|   stm32f401_d_e_ufbga100 IBIS Model
[IBIS ver]   4.2
[File name]  stm32f401_d_e_ufbga100.ibs
[File Rev]   1.0
[Date]   09-06-2015
[Source] Data Created at STMicroelectronics
[Notes]   File originated from ELDO simulations.
[Disclaimer]  This information is for modeling purpose only and is
   not guaranted. The information is subject to change without
   notice.
[Copyright] Copyright 2015 STMicroelectronics Inc.
[Component] stm32f401_d_e_ufbga100
[Manufacturer] STMicroelectronics
[Package]
| variable   typ   min   max
R_pkg   0.0   NA   NA
L_pkg   0.0H   NA   NA
C_pkg   0.0F   NA   NA
[Pin]   signal_name   model_name   R_pin   L_pin   C_pin
B2 PE2 io8p_arsudq_ft
A1 PE3 io8p_arsudq_ft
B1 PE4 io8p_arsudq_ft
C2 PE5 io8p_arsudq_ft
D2 PE6 io8p_arsudq_ft
D3 VSS GND
C4 VDD POWER
E2 VBAT POWER
C1 PC13-ANTI_TAMP io8p_arwsudq_ft_v33
D1 PC14-OSC32_IN io8p_arwsudq_ft
E1 PC15-OSC32_OUT io8p_arsudq_ft
F2 VSS GND
G2 VDD POWER
F1 PH0-OSC_IN io8p_arsudq_ft
G1 PH1-OSC_OUT io8p_arsudq_ft
H2 NRST ioreset_ft_v33
H1 PC0 io8p_arwsudq_ft
J2 PC1 io8p_arwsudq_ft
J3 PC2 io8p_arwsudq_ft
K2 PC3 io8p_arwsudq_ft
J1 VSSA GND
K1 VREF- GND
L1 VREF+ POWER
M1 VDDA POWER
L2 PA0-WKUP io8p_arwsudq_ft_v33
M2 PA1 io8p_arwsudq_ft
K3 PA2 io8p_arwsudq_ft
L3 PA3 io8p_arwsudq_ft
E3 BYPASS_REG NC
M3 PA4 io8p_ar3wsudq_ft
K4 PA5 io8p_ar3wsudq_ft
L4 PA6 io8p_ar3wsudq_ft
M4 PA7 io8p_arwsudq_ft
K5 PC4 io8p_arwsudq_ft
L5 PC5 io8p_arwsudq_ft
M5 PB0 io8p_ar3wsudq_ft
M6 PB1 io8p_ar3wsudq_ft
L6 PB2 io8p_arwsudq_ft
M7 PE7 io8p_arwsudq_ft
L7 PE8 io8p_arwsudq_ft
M8 PE9 io8p_arwsudq_ft
L8 PE10 io8p_arwsudq_ft
M9 PE11 io8p_arwsudq_ft
L9 PE12 io8p_arsudq_ft
M10 PE13 io8p_arsudq_ft
M11 PE14 io8p_arsudq_ft
M12 PE15 io8p_ar3wsudq_ft
L10 PB10 io8p_arsudq_i2cin_ft
K9 PB11 io8p_arsudq_ft
L11 VCAP1 POWER
F12 VSS GND
G12 VDD POWER
L12 PB12 io8p_arsudq_ft
K12 PB13 io8p_arsudq_ft
K11 PB14 io8p_arsudq_ft
K10 PB15 io8p_arsudq_ft
K8 PD9 io8p_arsudq_ft
J12 PD10 io8p_arsudq_ft
J11 PD11 io8p_arsudq_ft
J10 PD12 io8p_arsudq_ft
H12 PD13 io8p_arsudq_ft
H11 PD14 io8p_arsudq_ft
H10 PD15 io8p_arsudq_ft
E12 PC6 io8p_arsudq_ft
E11 PC7 io8p_arsudq_ft
E10 PC8 io8p_arsudq_ft
D12 PC9 io8p_arsudq_i2cin_ft
D11 PA8 io8p_arsudq_i2cin_ft
D10 PA9 io8usb_vbus_otg_ft
C12 PA10 io8usb_id_otg_ft
B12 PA11 io8usb_lsfs_otg_ft
A12 PA12 io8usb_lsfs_otg_ft
A11 PA13 io8p_arsudq_ft
C11 VCAP2 POWER
F11 VSS GND
G11 VDD POWER
A10 PA14 io8p_arsudq_ft
A9 PA15 io8p_arsudq_ft
B11 PC10 io8p_arsudq_ft
C10 PC11 io8p_arsudq_ft
B10 PC12 io8p_arsudq_ft
C9 PD0 io8p_arsudq_ft
B9 PD1 io8p_arsudq_ft
C8 PD2 io8p_arsudq_ft
B8 PD3 io8p_arsudq_ft
B7 PD4 io8p_arsudq_ft
A6 PD5 io8p_arsudq_ft
B6 PD6 io8p_arsudq_ft
A5 PD7 io8p_arsudq_ft
A8 PB3 io8p_arsudq_i2cin_ft
A7 PB4 io8p_arsudq_i2cin_ft
C5 PB5 io8p_ar3wsudq_ft
B5 PB6 io8p_arsudq_i2cin_ft
B4 PB7 io8p_arsudq_i2cin_ft
A4 BOOT0 vpp_test_hv
A3 PB8 io8p_arsudq_i2cin_ft
B3 PB9 io8p_arsudq_i2cin_ft
C3 PE0 io8p_arsudq_ft
A2 PE1 io8p_arsudq_ft
H3 PDR_ON NC
[Diff Pin]   inv_pin   vdiff   tdelay_typ  tdelay_min  tdelay_max
B12 A12 200mV   NA   NA   NA
[Model Selector] io8p_ar3wsudq_ft
io8p00_ar3wsudq_ft_pd_lv  "SPEED00 1P8V, PD=40kOhm"
io8p00_ar3wsudq_ft_pu_lv  "SPEED00 1P8V, PU=40kOhm"
io8p00_ar3wsudq_ft_lv  "SPEED00 1P8V"
io8p01_ar3wsudq_ft_pd_lv  "SPEED01 1P8V, PD=40kOhm"
io8p01_ar3wsudq_ft_pu_lv  "SPEED01 1P8V, PU=40kOhm"
io8p01_ar3wsudq_ft_lv  "SPEED01 1P8V"
io8p10_ar3wsudq_ft_pd_lv  "SPEED10 1P8V, PD=40kOhm"
io8p10_ar3wsudq_ft_pu_lv  "SPEED10 1P8V, PU=40kOhm"
io8p10_ar3wsudq_ft_lv  "SPEED10 1P8V"
io8p11_ar3wsudq_ft_pd_lv  "SPEED11 1P8V, PD=40kOhm"
io8p11_ar3wsudq_ft_pu_lv  "SPEED11 1P8V, PU=40kOhm"
io8p11_ar3wsudq_ft_lv  "SPEED11 1P8V"
io8p00_ar3wsudq_ft_pd  "SPEED00, PD=40kOhm"
io8p00_ar3wsudq_ft_pu  "SPEED00, PU=40kOhm"
io8p00_ar3wsudq_ft  "SPEED00"
io8p01_ar3wsudq_ft_pd  "SPEED01, PD=40kOhm"
io8p01_ar3wsudq_ft_pu  "SPEED01, PU=40kOhm"
io8p01_ar3wsudq_ft  "SPEED01"
io8p10_ar3wsudq_ft_pd  "SPEED10, PD=40kOhm"
io8p10_ar3wsudq_ft_pu  "SPEED10, PU=40kOhm"
io8p10_ar3wsudq_ft  "SPEED10"
io8p11_ar3wsudq_ft_pd  "SPEED11, PD=40kOhm"
io8p11_ar3wsudq_ft_pu  "SPEED11, PU=40kOhm"
io8p11_ar3wsudq_ft  "SPEED11"
[Model Selector] io8p_arsudq_ft
io8p00_arsudq_ft_pd_lv  "SPEED00 1P8V, PD=40kOhm"
io8p00_arsudq_ft_pu_lv  "SPEED00 1P8V, PU=40kOhm"
io8p00_arsudq_ft_lv  "SPEED00 1P8V"
io8p01_arsudq_ft_pd_lv  "SPEED01 1P8V, PD=40kOhm"
io8p01_arsudq_ft_pu_lv  "SPEED01 1P8V, PU=40kOhm"
io8p01_arsudq_ft_lv  "SPEED01 1P8V"
io8p10_arsudq_ft_pd_lv  "SPEED10 1P8V, PD=40kOhm"
io8p10_arsudq_ft_pu_lv  "SPEED10 1P8V, PU=40kOhm"
io8p10_arsudq_ft_lv  "SPEED10 1P8V"
io8p11_arsudq_ft_pd_lv  "SPEED11 1P8V, PD=40kOhm"
io8p11_arsudq_ft_pu_lv  "SPEED11 1P8V, PU=40kOhm"
io8p11_arsudq_ft_lv  "SPEED11 1P8V"
io8p00_arsudq_ft_pd  "SPEED00, PD=40kOhm"
io8p00_arsudq_ft_pu  "SPEED00, PU=40kOhm"
io8p00_arsudq_ft  "SPEED00"
io8p01_arsudq_ft_pd  "SPEED01, PD=40kOhm"
io8p01_arsudq_ft_pu  "SPEED01, PU=40kOhm"
io8p01_arsudq_ft  "SPEED01"
io8p10_arsudq_ft_pd  "SPEED10, PD=40kOhm"
io8p10_arsudq_ft_pu  "SPEED10, PU=40kOhm"
io8p10_arsudq_ft  "SPEED10"
io8p11_arsudq_ft_pd  "SPEED11, PD=40kOhm"
io8p11_arsudq_ft_pu  "SPEED11, PU=40kOhm"
io8p11_arsudq_ft  "SPEED11"
[Model Selector] io8p_arsudq_i2cin_ft
io8p00_arsudq_i2cin_ft_pd_lv  "SPEED00 1P8V, PD=40kOhm"
io8p00_arsudq_i2cin_ft_pu_lv  "SPEED00 1P8V, PU=40kOhm"
io8p00_arsudq_i2cin_ft_lv  "SPEED00 1P8V"
io8p01_arsudq_i2cin_ft_pd_lv  "SPEED01 1P8V, PD=40kOhm"
io8p01_arsudq_i2cin_ft_pu_lv  "SPEED01 1P8V, PU=40kOhm"
io8p01_arsudq_i2cin_ft_lv  "SPEED01 1P8V"
io8p10_arsudq_i2cin_ft_pd_lv  "SPEED10 1P8V, PD=40kOhm"
io8p10_arsudq_i2cin_ft_pu_lv  "SPEED10 1P8V, PU=40kOhm"
io8p10_arsudq_i2cin_ft_lv  "SPEED10 1P8V"
io8p11_arsudq_i2cin_ft_pd_lv  "SPEED11 1P8V, PD=40kOhm"
io8p11_arsudq_i2cin_ft_pu_lv  "SPEED11 1P8V, PU=40kOhm"
io8p11_arsudq_i2cin_ft_lv  "SPEED11 1P8V"
io8p00_arsudq_i2cin_ft_pd  "SPEED00, PD=40kOhm"
io8p00_arsudq_i2cin_ft_pu  "SPEED00, PU=40kOhm"
io8p00_arsudq_i2cin_ft  "SPEED00"
io8p01_arsudq_i2cin_ft_pd  "SPEED01, PD=40kOhm"
io8p01_arsudq_i2cin_ft_pu  "SPEED01, PU=40kOhm"
io8p01_arsudq_i2cin_ft  "SPEED01"
io8p10_arsudq_i2cin_ft_pd  "SPEED10, PD=40kOhm"
io8p10_arsudq_i2cin_ft_pu  "SPEED10, PU=40kOhm"
io8p10_arsudq_i2cin_ft  "SPEED10"
io8p11_arsudq_i2cin_ft_pd  "SPEED11, PD=40kOhm"
io8p11_arsudq_i2cin_ft_pu  "SPEED11, PU=40kOhm"
io8p11_arsudq_i2cin_ft  "SPEED11"
[Model Selector] io8p_arwsudq_ft
io8p00_arwsudq_ft_pd_lv  "SPEED00 1P8V, PD=40kOhm"
io8p00_arwsudq_ft_pu_lv  "SPEED00 1P8V, PU=40kOhm"
io8p00_arwsudq_ft_lv  "SPEED00 1P8V"
io8p01_arwsudq_ft_pd_lv  "SPEED01 1P8V, PD=40kOhm"
io8p01_arwsudq_ft_pu_lv  "SPEED01 1P8V, PU=40kOhm"
io8p01_arwsudq_ft_lv  "SPEED01 1P8V"
io8p10_arwsudq_ft_pd_lv  "SPEED10 1P8V, PD=40kOhm"
io8p10_arwsudq_ft_pu_lv  "SPEED10 1P8V, PU=40kOhm"
io8p10_arwsudq_ft_lv  "SPEED10 1P8V"
io8p11_arwsudq_ft_pd_lv  "SPEED11 1P8V, PD=40kOhm"
io8p11_arwsudq_ft_pu_lv  "SPEED11 1P8V, PU=40kOhm"
io8p11_arwsudq_ft_lv  "SPEED11 1P8V"
io8p00_arwsudq_ft_pd  "SPEED00, PD=40kOhm"
io8p00_arwsudq_ft_pu  "SPEED00, PU=40kOhm"
io8p00_arwsudq_ft  "SPEED00"
io8p01_arwsudq_ft_pd  "SPEED01, PD=40kOhm"
io8p01_arwsudq_ft_pu  "SPEED01, PU=40kOhm"
io8p01_arwsudq_ft  "SPEED01"
io8p10_arwsudq_ft_pd  "SPEED10, PD=40kOhm"
io8p10_arwsudq_ft_pu  "SPEED10, PU=40kOhm"
io8p10_arwsudq_ft  "SPEED10"
io8p11_arwsudq_ft_pd  "SPEED11, PD=40kOhm"
io8p11_arwsudq_ft_pu  "SPEED11, PU=40kOhm"
io8p11_arwsudq_ft  "SPEED11"
[Model Selector] io8p_arwsudq_ft_v33
io8p00_arwsudq_ft_v33_pd_lv  "SPEED00 1P8V, PD=40kOhm"
io8p00_arwsudq_ft_v33_pu_lv  "SPEED00 1P8V, PU=40kOhm"
io8p00_arwsudq_ft_v33_lv  "SPEED00 1P8V"
io8p01_arwsudq_ft_v33_pd_lv  "SPEED01 1P8V, PD=40kOhm"
io8p01_arwsudq_ft_v33_pu_lv  "SPEED01 1P8V, PU=40kOhm"
io8p01_arwsudq_ft_v33_lv  "SPEED01 1P8V"
io8p10_arwsudq_ft_v33_pd_lv  "SPEED10 1P8V, PD=40kOhm"
io8p10_arwsudq_ft_v33_pu_lv  "SPEED10 1P8V, PU=40kOhm"
io8p10_arwsudq_ft_v33_lv  "SPEED10 1P8V"
io8p11_arwsudq_ft_v33_pd_lv  "SPEED11 1P8V, PD=40kOhm"
io8p11_arwsudq_ft_v33_pu_lv  "SPEED11 1P8V, PU=40kOhm"
io8p11_arwsudq_ft_v33_lv  "SPEED11 1P8V"
io8p00_arwsudq_ft_v33_pd  "SPEED00, PD=40kOhm"
io8p00_arwsudq_ft_v33_pu  "SPEED00, PU=40kOhm"
io8p00_arwsudq_ft_v33  "SPEED00"
io8p01_arwsudq_ft_v33_pd  "SPEED01, PD=40kOhm"
io8p01_arwsudq_ft_v33_pu  "SPEED01, PU=40kOhm"
io8p01_arwsudq_ft_v33  "SPEED01"
io8p10_arwsudq_ft_v33_pd  "SPEED10, PD=40kOhm"
io8p10_arwsudq_ft_v33_pu  "SPEED10, PU=40kOhm"
io8p10_arwsudq_ft_v33  "SPEED10"
io8p11_arwsudq_ft_v33_pd  "SPEED11, PD=40kOhm"
io8p11_arwsudq_ft_v33_pu  "SPEED11, PU=40kOhm"
io8p11_arwsudq_ft_v33  "SPEED11"
[Model Selector] io8usb_id_otg_ft
io8p00_id_otg_ft_pd_lv  "SPEED00 1P8V, PD=14kOhm"
io8p00_id_otg_ft_pu_lv  "SPEED00 1P8V, PU=14kOhm"
io8p00_id_otg_ft_lv  "SPEED00 1P8V"
io8p01_id_otg_ft_pd_lv  "SPEED01 1P8V, PD=14kOhm"
io8p01_id_otg_ft_pu_lv  "SPEED01 1P8V, PU=14kOhm"
io8p01_id_otg_ft_lv  "SPEED01 1P8V"
io8p10_id_otg_ft_pd_lv  "SPEED10 1P8V, PD=14kOhm"
io8p10_id_otg_ft_pu_lv  "SPEED10 1P8V, PU=14kOhm"
io8p10_id_otg_ft_lv  "SPEED10 1P8V"
io8p11_id_otg_ft_pd_lv  "SPEED11 1P8V, PD=14kOhm"
io8p11_id_otg_ft_pu_lv  "SPEED11 1P8V, PU=14kOhm"
io8p11_id_otg_ft_lv  "SPEED11 1P8V"
io8p00_id_otg_ft_pd  "SPEED00, PD=14kOhm"
io8p00_id_otg_ft_pu  "SPEED00, PU=14kOhm"
io8p00_id_otg_ft  "SPEED00"
io8p01_id_otg_ft_pd  "SPEED01, PD=14kOhm"
io8p01_id_otg_ft_pu  "SPEED01, PU=14kOhm"
io8p01_id_otg_ft  "SPEED01"
io8p10_id_otg_ft_pd  "SPEED10, PD=14kOhm"
io8p10_id_otg_ft_pu  "SPEED10, PU=14kOhm"
io8p10_id_otg_ft  "SPEED10"
io8p11_id_otg_ft_pd  "SPEED11, PD=14kOhm"
io8p11_id_otg_ft_pu  "SPEED11, PU=14kOhm"
io8p11_id_otg_ft  "SPEED11"
[Model Selector] io8usb_lsfs_otg_ft
io8usb_ls_otg_ft_dpdn_pd  "LS USB DP/DN IO + PD=20kOhm"
io8usb_ls_otg_ft_dpdn_pupu2  "LS USB DP/DN IO + PU/PU2=2.2kOhm"
io8usb_ls_otg_ft_dpdn_pu2  "LS USB DP/DN IO + PU2=1.2kOhm"
io8usb_ls_otg_ft_dpdn_pu  "LS USB DP/DN IO + PU=1.2kOhm"
io8usb_ls_otg_ft_dpdn  "LS USB DP/DN IO"
io8usb_fs_otg_ft_dpdn_pd  "HS USB DP/DN IO + PD=20kOhm"
io8usb_fs_otg_ft_dpdn_pupu2  "HS USB DP/DN IO + PU/PU2=2.2kOhm"
io8usb_fs_otg_ft_dpdn_pu2  "HS USB DP/DN IO + PU2=1.2kOhm"
io8usb_fs_otg_ft_dpdn_pu  "HS USB DP/DN IO + PU=1.2kOhm"
io8usb_fs_otg_ft_dpdn  "HS USB DP/DN IO"
io8p00_lsfs_otg_ft_pd_lv  "SPEED00 1P8V, PD=40kOhm"
io8p00_lsfs_otg_ft_pu_lv  "SPEED00 1P8V, PU=40kOhm"
io8p00_lsfs_otg_ft_lv  "SPEED00 1P8V"
io8p01_lsfs_otg_ft_pd_lv  "SPEED01 1P8V, PD=40kOhm"
io8p01_lsfs_otg_ft_pu_lv  "SPEED01 1P8V, PU=40kOhm"
io8p01_lsfs_otg_ft_lv  "SPEED01 1P8V"
io8p10_lsfs_otg_ft_pd_lv  "SPEED10 1P8V, PD=40kOhm"
io8p10_lsfs_otg_ft_pu_lv  "SPEED10 1P8V, PU=40kOhm"
io8p10_lsfs_otg_ft_lv  "SPEED10 1P8V"
io8p11_lsfs_otg_ft_pd_lv  "SPEED11 1P8V, PD=40kOhm"
io8p11_lsfs_otg_ft_pu_lv  "SPEED11 1P8V, PU=40kOhm"
io8p11_lsfs_otg_ft_lv  "SPEED11 1P8V"
io8p00_lsfs_otg_ft_pd  "SPEED00, PD=40kOhm"
io8p00_lsfs_otg_ft_pu  "SPEED00, PU=40kOhm"
io8p00_lsfs_otg_ft  "SPEED00"
io8p01_lsfs_otg_ft_pd  "SPEED01, PD=40kOhm"
io8p01_lsfs_otg_ft_pu  "SPEED01, PU=40kOhm"
io8p01_lsfs_otg_ft  "SPEED01"
io8p10_lsfs_otg_ft_pd  "SPEED10, PD=40kOhm"
io8p10_lsfs_otg_ft_pu  "SPEED10, PU=40kOhm"
io8p10_lsfs_otg_ft  "SPEED10"
io8p11_lsfs_otg_ft_pd  "SPEED11, PD=40kOhm"
io8p11_lsfs_otg_ft_pu  "SPEED11, PU=40kOhm"
io8p11_lsfs_otg_ft  "SPEED11"
[Model Selector] io8usb_vbus_otg_ft
io8psenb_vbus_otg_ft  "VBUS PULSE, SENSE VB"
io8psenab_vbus_otg_ft  "VBUS PULSE, SENSE VA and VB"
io8psena_vbus_otg_ft  "VBUS PULSE, SENSE VA"
io8psen_vbus_otg_ft  "VBUS PULSE"
io8p00_vbus_otg_ft_pd_lv  "SPEED00 1P8V, PD=40kOhm"
io8p00_vbus_otg_ft_pu_lv  "SPEED00 1P8V, PU=40kOhm"
io8p00_vbus_otg_ft_lv  "SPEED00 1P8V"
io8p01_vbus_otg_ft_pd_lv  "SPEED01 1P8V, PD=40kOhm"
io8p01_vbus_otg_ft_pu_lv  "SPEED01 1P8V, PU=40kOhm"
io8p01_vbus_otg_ft_lv  "SPEED01 1P8V"
io8p10_vbus_otg_ft_pd_lv  "SPEED10 1P8V, PD=40kOhm"
io8p10_vbus_otg_ft_pu_lv  "SPEED10 1P8V, PU=40kOhm"
io8p10_vbus_otg_ft_lv  "SPEED10 1P8V"
io8p11_vbus_otg_ft_pd_lv  "SPEED11 1P8V, PD=40kOhm"
io8p11_vbus_otg_ft_pu_lv  "SPEED11 1P8V, PU=40kOhm"
io8p11_vbus_otg_ft_lv  "SPEED11 1P8V"
io8p00_vbus_otg_ft_pd  "SPEED00, PD=40kOhm"
io8p00_vbus_otg_ft_pu  "SPEED00, PU=40kOhm"
io8p00_vbus_otg_ft  "SPEED00"
io8p01_vbus_otg_ft_pd  "SPEED01, PD=40kOhm"
io8p01_vbus_otg_ft_pu  "SPEED01, PU=40kOhm"
io8p01_vbus_otg_ft  "SPEED01"
io8p10_vbus_otg_ft_pd  "SPEED10, PD=40kOhm"
io8p10_vbus_otg_ft_pu  "SPEED10, PU=40kOhm"
io8p10_vbus_otg_ft  "SPEED10"
io8p11_vbus_otg_ft_pd  "SPEED11, PD=40kOhm"
io8p11_vbus_otg_ft_pu  "SPEED11, PU=40kOhm"
io8p11_vbus_otg_ft  "SPEED11"
[Model Selector] ioreset_ft_v33
ioreset_ft_v33_pu_lv  "ioreset 1P8V + PU=40kOhm"
ioreset_ft_v33_nopu_lv  "ioreset 1P8V"
ioreset_ft_v33_pu  "ioreset + PU=40kOhm"
ioreset_ft_v33_nopu  "ioreset"
[Model Selector] vpp_test_hv
vpp_test_hv_2p4  "Input Buffer 1P8V"
vpp_test_hv_3p3  "Input Buffer"
| Models and submodels in the file (212): io8p00_ar3wsudq_ft_pd_lv (I/O), io8p00_ar3wsudq_ft_pu_lv (I/O), io8p00_ar3wsudq_ft_lv (I/O), io8p01_ar3wsudq_ft_pd_lv (I/O), io8p01_ar3wsudq_ft_pu_lv (I/O), io8p01_ar3wsudq_ft_lv (I/O), io8p10_ar3wsudq_ft_pd_lv (I/O), io8p10_ar3wsudq_ft_pu_lv (I/O), io8p10_ar3wsudq_ft_lv (I/O), io8p11_ar3wsudq_ft_pd_lv (I/O), io8p11_ar3wsudq_ft_pu_lv (I/O), io8p11_ar3wsudq_ft_lv (I/O), io8p00_ar3wsudq_ft_pd (I/O), io8p00_ar3wsudq_ft_pu (I/O), io8p00_ar3wsudq_ft (I/O), io8p01_ar3wsudq_ft_pd (I/O), io8p01_ar3wsudq_ft_pu (I/O), io8p01_ar3wsudq_ft (I/O), io8p10_ar3wsudq_ft_pd (I/O), io8p10_ar3wsudq_ft_pu (I/O), io8p10_ar3wsudq_ft (I/O), io8p11_ar3wsudq_ft_pd (I/O), io8p11_ar3wsudq_ft_pu (I/O), io8p11_ar3wsudq_ft (I/O), io8p00_arsudq_ft_pd_lv (I/O), io8p00_arsudq_ft_pu_lv (I/O), io8p00_arsudq_ft_lv (I/O), io8p01_arsudq_ft_pd_lv (I/O), io8p01_arsudq_ft_pu_lv (I/O), io8p01_arsudq_ft_lv (I/O), io8p10_arsudq_ft_pd_lv (I/O), io8p10_arsudq_ft_pu_lv (I/O), io8p10_arsudq_ft_lv (I/O), io8p11_arsudq_ft_pd_lv (I/O), io8p11_arsudq_ft_pu_lv (I/O), io8p11_arsudq_ft_lv (I/O), io8p00_arsudq_ft_pd (I/O), io8p00_arsudq_ft_pu (I/O), io8p00_arsudq_ft (I/O), io8p01_arsudq_ft_pd (I/O), io8p01_arsudq_ft_pu (I/O), io8p01_arsudq_ft (I/O), io8p10_arsudq_ft_pd (I/O), io8p10_arsudq_ft_pu (I/O), io8p10_arsudq_ft (I/O), io8p11_arsudq_ft_pd (I/O), io8p11_arsudq_ft_pu (I/O), io8p11_arsudq_ft (I/O), io8p00_arsudq_i2cin_ft_pd_lv (I/O), io8p00_arsudq_i2cin_ft_pu_lv (I/O), io8p00_arsudq_i2cin_ft_lv (I/O), io8p01_arsudq_i2cin_ft_pd_lv (I/O), io8p01_arsudq_i2cin_ft_pu_lv (I/O), io8p01_arsudq_i2cin_ft_lv (I/O), io8p10_arsudq_i2cin_ft_pd_lv (I/O), io8p10_arsudq_i2cin_ft_pu_lv (I/O), io8p10_arsudq_i2cin_ft_lv (I/O), io8p11_arsudq_i2cin_ft_pd_lv (I/O), io8p11_arsudq_i2cin_ft_pu_lv (I/O), io8p11_arsudq_i2cin_ft_lv (I/O), io8p00_arsudq_i2cin_ft_pd (I/O), io8p00_arsudq_i2cin_ft_pu (I/O), io8p00_arsudq_i2cin_ft (I/O), io8p01_arsudq_i2cin_ft_pd (I/O), io8p01_arsudq_i2cin_ft_pu (I/O), io8p01_arsudq_i2cin_ft (I/O), io8p10_arsudq_i2cin_ft_pd (I/O), io8p10_arsudq_i2cin_ft_pu (I/O), io8p10_arsudq_i2cin_ft (I/O), io8p11_arsudq_i2cin_ft_pd (I/O), io8p11_arsudq_i2cin_ft_pu (I/O), io8p11_arsudq_i2cin_ft (I/O), io8p00_arwsudq_ft_pd_lv (I/O), io8p00_arwsudq_ft_pu_lv (I/O), io8p00_arwsudq_ft_lv (I/O), io8p01_arwsudq_ft_pd_lv (I/O), io8p01_arwsudq_ft_pu_lv (I/O), io8p01_arwsudq_ft_lv (I/O), io8p10_arwsudq_ft_pd_lv (I/O), io8p10_arwsudq_ft_pu_lv (I/O)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
